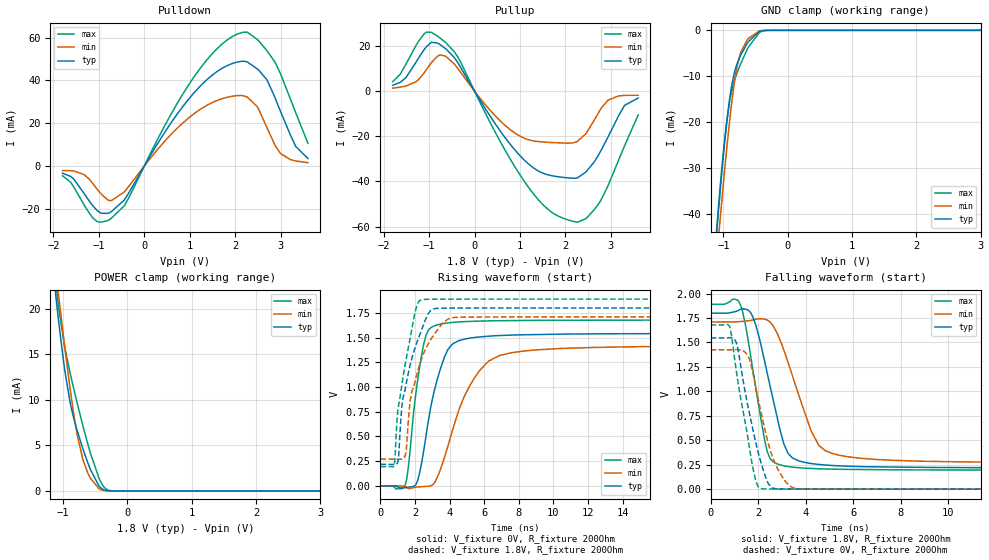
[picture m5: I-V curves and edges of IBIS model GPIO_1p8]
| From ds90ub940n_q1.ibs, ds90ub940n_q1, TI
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|   Model
[Model]   GPIO_1p8
Model_type   I/O
Polarity   Non-Inverting
Enable   Active-Low
Vinl = 0.63
Vinh = 1.17
Vmeas = 0.9
Vref = 0
Cref = 1pF
Rref = 10000
|   typ   min   max
C_comp   1.5999pF   1.5084pF   1.9148pF
[Voltage Range]   1.8   1.71   1.89
[Temperature Range]   27   105   -40
[Pullup Reference]   1.8   1.71   1.89
[Pulldown Reference]   0   0   -0
[Power Clamp Reference]   1.8   1.71   1.89
[GND Clamp Reference]   0   0   0
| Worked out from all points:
|   slope of the pulldown table from 0 to 0.27 V, typ, clamps not added: 27.8 ohm
|   slope of the pullup table from 0 to 0.27 V, typ, clamps not added: 30.7 ohm
|   GND clamp passes 1 mA (typ) near -0.50 V on its own axis
|   POWER clamp passes 1 mA (typ) near -0.48 V on its own axis
|   falling waveform, V_fixture 1.8V, R_fixture 200Ohm: 20-80 % time 890ps typ, 1.23ns min, 687ps max; typ from 1.8 V to 0.218 V
|   rising waveform, V_fixture 0V, R_fixture 200Ohm: 20-80 % time 1.11ns typ, 1.93ns min, 703ps max; typ from 0 V to 1.55 V
|   rising waveform, V_fixture 1.8V, R_fixture 200Ohm: 20-80 % time 1.05ns typ, 1.15ns min, 864ps max; typ from 0.218 V to 1.8 V
|   falling waveform, V_fixture 0V, R_fixture 200Ohm: 20-80 % time 793ps typ, 859ps min, 687ps max; typ from 1.55 V to 0 V
[Pulldown]
|   Voltage   I(typ)   I(min)   I(max)
-1.8V     -3.442mA   -2.153mA   -4.619mA
-1.552V   -6.211mA   -2.4mA     -9.905mA
-1.136V   -18.61mA   -8.197mA   -24.27mA
-730.8mV  -21.48mA   -16.27mA   -24.56mA
-444.6mV  -16.05mA   -12.26mA   -18.74mA
1.143V    35.4mA     25.22mA    43.19mA
1.737V    46.03mA    31.66mA    57.54mA
2.201V    48.99mA    32.73mA    62.65mA
2.482V    45.47mA    27.76mA    59.28mA
2.893V    30.91mA    9.011mA    47.8mA
3.33V     9.124mA    2.31mA     24.89mA
3.6V      3.451mA    1.52mA     10.56mA
[GND Clamp]
|   Voltage   I(typ)   I(min)   I(max)
-1.8V     -180.4mA   -173.5mA   -189.7mA
-1.109V   -44.75mA   -50.41mA   -43.86mA
-1.076V   -39.18mA   -45.13mA   -38.17mA
-1.033V   -32.1mA    -38.28mA   -31.16mA
-963mV    -21.82mA   -27.73mA   -21.52mA
-914.4mV  -15.99mA   -21.04mA   -16.41mA
-876.6mV  -12.4mA    -16.33mA   -13.49mA
-790.2mV  -7.348mA   -8.022mA   -9.368mA
-736.2mV  -5.494mA   -4.97mA    -7.431mA
-633.6mV  -2.91mA    -2.134mA   -4.217mA
-444.6mV  -246uA     -153.4uA   -518.5uA
3.6V      0A         0A         0A
[Pullup]
|   Voltage   I(typ)   I(min)   I(max)
-1.8V     2.589mA    1.353mA    4.195mA
-1.508V   6.003mA    2.254mA    11.95mA
-1.114V   18.24mA    7.945mA    25.27mA
-752.4mV  20.53mA    16.02mA    23.43mA
-369mV    12.62mA    10.07mA    15.16mA
462.6mV   -14.68mA   -11.09mA   -18.45mA
1.084V    -30.31mA   -20.75mA   -39.62mA
1.672V    -37.34mA   -22.73mA   -53.25mA
2.255V    -38.44mA   -22.29mA   -58.01mA
2.758V    -27.16mA   -8.518mA   -49.1mA
3.303V    -6.264mA   -1.868mA   -24.11mA
3.6V      -3.073mA   -1.832mA   -10.54mA
[POWER Clamp]
|   Voltage   I(typ)   I(min)   I(max)
-1.8V     70.84mA    69.22mA    78.42mA
-1.179V   25.69mA    28.2mA     27.24mA
-1.098V   20.36mA    23.14mA    21.79mA
-1.071V   18.66mA    21.48mA    20.2mA
-973.8mV  13.18mA    15.72mA    15.73mA
-892.8mV  9.749mA    11.27mA    12.99mA
-779.4mV  6.564mA    6.099mA    9.577mA
-693mV    4.627mA    3.454mA    7.149mA
-617.4mV  3.111mA    1.993mA    5.166mA
-428.4mV  441.2uA    196.1uA    1.193mA
-217.8mV  1.765uA    1.343uA    8.112uA
3.6V      0A         0A         0A
[Ramp]
R_load = 200
|   typ   min   max
dV/dt_r   0.927493/1.11309e-09   0.855131/1.93106e-09   1.00756/7.02651e-10
dV/dt_f   0.949023/8.90457e-10   0.863713/1.22897e-09   1.01683/6.87274e-10
[Falling Waveform]
V_fixture = 1.8V
V_fixture_min = 1.71V
V_fixture_max = 1.89V
R_fixture = 200Ohm
C_fixture = 0F
|   Time   V(typ)   V(min)   V(max)
0s        1.8V       1.71V      1.89V
1.165ns   1.828V     1.712V     1.926V
1.444ns   1.841V     1.719V     1.707V
1.692ns   1.802V     1.726V     1.352V
2.375ns   1.193V     1.73V      388.7mV
3.111ns   445.8mV    1.401V     237.2mV
3.44ns    319.6mV    1.16V      225.6mV
4.547ns   252.9mV    449.3mV    208.4mV
6.246ns   231.8mV    317.3mV    201.2mV
40ns      218.3mV    270.5mV    195.3mV
[Rising Waveform]
V_fixture = 0V
V_fixture_min = 0V
V_fixture_max = 0V
R_fixture = 200Ohm
C_fixture = 0F
|   Time   V(typ)   V(min)   V(max)
0s        9.743uV    449.1nV    2.198uV
1.444ns   -16.43mV   -9.664mV   12.84mV
1.599ns   -12.54mV   -26mV      169.8mV
2.043ns   10.46mV    -13.2mV    928.1mV
2.502ns   357.7mV    -6.419mV   1.434V
3.306ns   1.089V     94.29mV    1.631V
4.154ns   1.434V     555mV      1.653V
5.401ns   1.5V       1.083V     1.666V
7.581ns   1.526V     1.347V     1.672V
40ns      1.546V     1.425V     1.679V
[Rising Waveform]
V_fixture = 1.8V
V_fixture_min = 1.71V
V_fixture_max = 1.89V
R_fixture = 200Ohm
C_fixture = 0F
|   Time   V(typ)   V(min)   V(max)
0s        218.3mV    270.5mV    195.2mV
803.1ps   217.3mV    270.3mV    216.2mV
1.034ns   269.1mV    270.2mV    800mV
1.221ns   773.3mV    270.2mV    1.002V
1.398ns   953.1mV    292.5mV    1.195V
1.792ns   1.275V     937mV      1.564V
2.375ns   1.576V     1.283V     1.884V
2.909ns   1.776V     1.48V      1.888V
4.547ns   1.799V     1.707V     1.889V
40ns      1.8V       1.71V      1.89V
[Falling Waveform]
|Gnd
V_fixture = 0V
V_fixture_min = 0V
V_fixture_max = 0V
R_fixture = 200Ohm
C_fixture = 0F
|   Time   V(typ)   V(min)   V(max)
0s        1.547V     1.425V     1.68V
815.1ps   1.549V     1.425V     1.653V
1.113ns   1.474V     1.427V     1.157V
1.575ns   842.3mV    1.36V      511.3mV
1.908ns   467.8mV    1.032V     76.01mV
2.126ns   266.4mV    782.2mV    5.742mV
2.43ns    54.86mV    466.4mV    1.767mV
2.813ns   3.219mV    210.5mV    975.7uV
3.663ns   1.65mV     5.168mV    642uV
40ns      8.045uV    449.1nV    10.28uV
